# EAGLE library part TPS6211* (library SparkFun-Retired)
TPS62112: 1.5A Step-Down Converter
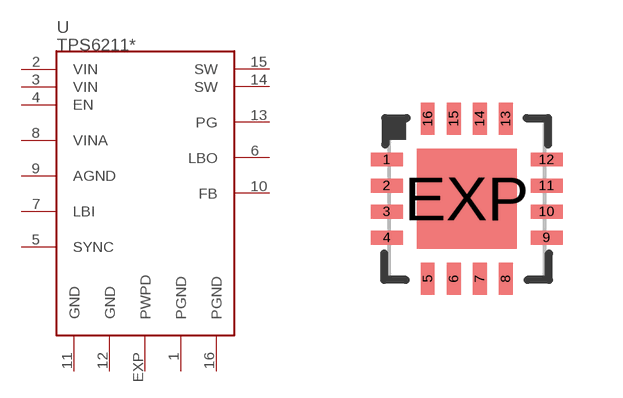
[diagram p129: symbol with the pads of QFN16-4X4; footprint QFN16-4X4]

Designator prefix U

## TPS6211  [QFN16-4X4]
1  PGND  pwr
2  VIN  pwr
3  VIN  pwr
4  EN  in
5  SYNC  in
6  LBO  out
7  LBI  in
8  VINA  pwr
9  AGND  pwr
10  FB  in
11  GND  pwr
12  GND  pwr
13  PG  out
14  SW  out
15  SW  out
16  PGND  pwr
EXP  PWPD  pwr

## Footprint QFN16-4X4 (pad centres in mm)
16-Lead Plastic Quad Flat, No Lead Package (ML) - 4x4x0.9mm Body [QFN] Source: http://ww1.microchip.com/downloads/en/DeviceDoc/41203E.pdf
smd 0.8 x 0.35: 1 -2,0.975; 2 -2,0.325; 3 -2,-0.325; 4 -2,-0.975; 9 2,-0.975; 10 2,-0.325; 11 2,0.325; 12 2,0.975
smd 0.35 x 0.8: 5 -0.975,-2; 6 -0.325,-2; 7 0.325,-2; 8 0.975,-2; 13 0.975,2; 14 0.325,2; 15 -0.325,2; 16 -0.975,2
smd 2.5 x 2.5: EXP 0,0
